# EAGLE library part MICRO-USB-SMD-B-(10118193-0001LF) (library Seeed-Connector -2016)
320010003
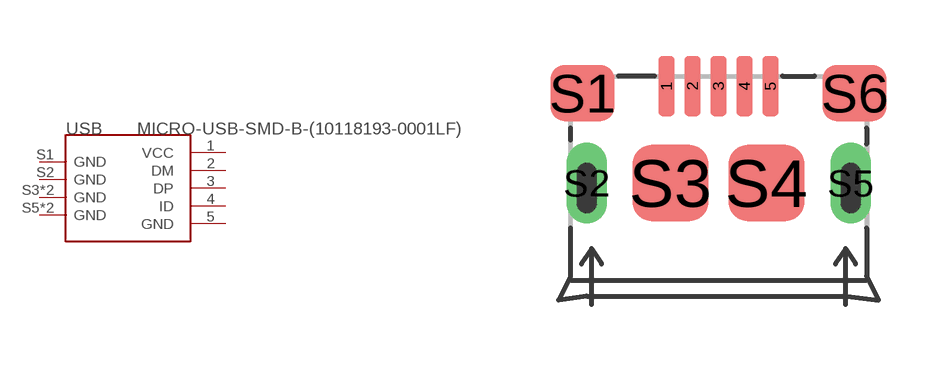
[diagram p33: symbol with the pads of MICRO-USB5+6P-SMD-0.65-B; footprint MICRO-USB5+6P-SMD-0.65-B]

Designator prefix USB

## MICRO-USB-SMD-B-(10118193-0001LF) (MPN: 10118193-0001LF; VALUE: 10118193-0001LF)  [MICRO-USB5+6P-SMD-0.65-B]
1  VCC
2  DM
3  DP
4  ID
5  GND
S1  GND
S2  GND
S3  GND
S4  GND
S5  GND
S6  GND

## Footprint MICRO-USB5+6P-SMD-0.65-B (pad centres in mm)
smd 0.4 x 1.5: 1 -1.3,-0.25; 2 -0.65,-0.25; 3 0,-0.25; 4 0.65,-0.25; 5 1.3,-0.25
smd 1.6 x 1.4: S1 -3.4,-0.427; S6 3.4,-0.427
drill 0.508 pad 1.016 long: S2 -3.3,-2.675; S5 3.3,-2.675
smd 1.9 x 1.9: S3 -1.2,-2.675; S4 1.2,-2.675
